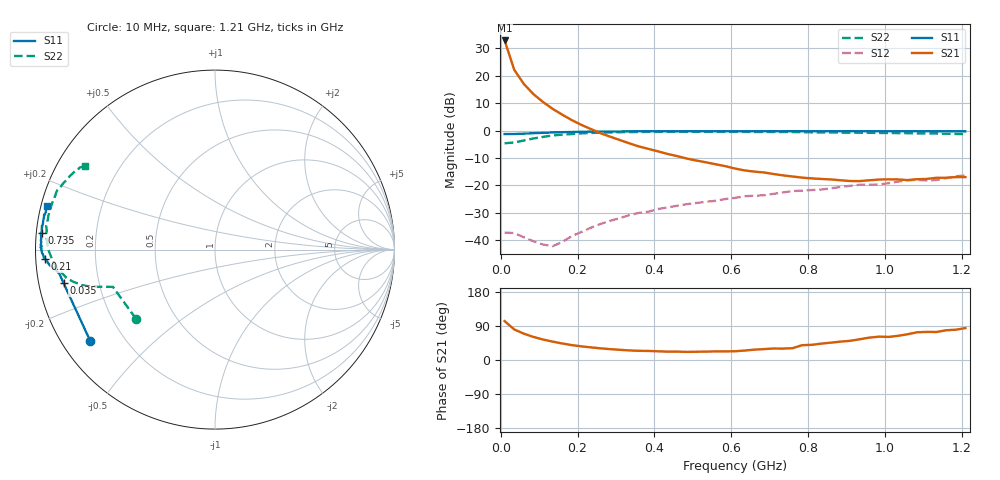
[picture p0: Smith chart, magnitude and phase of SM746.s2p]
!  POLYFET RF DEVICES
!  SM746
!  S PARAMETERS
!  VDS=50V, IDQ=600mA
# MHZ S MA R 50
! Freq=Mhz Mag[s11] Ang[s11] Mag[s21] Ang[s21] Mag[s12] Ang[s12] Mag[s22] Ang[s22]
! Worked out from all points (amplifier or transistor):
!   49 points, 10 MHz to 1.21 GHz, reference 50 ohm
!   highest |S21| = 32.8 dB at 10 MHz (marker M1)
!   |S21| within 3 dB of that: start of sweep to 17.04 MHz
!   unconditionally stable (mu >= 1): 121.7 MHz to 173.5 MHz; 679.3 MHz to end of sweep
!   at 210 MHz: K = 0.84, MSG = 19.5 dB, |S12| = -36.9 dB
!   at 610 MHz: K = 0.88, MSG = 5.3 dB, |S12| = -24.5 dB
!   at 1.21 GHz: K = 1.04, MAG = -1.6 dB, |S12| = -16.3 dB
!   S11 on the Smith chart (normalised r, x): 10 MHz: 0.08, -0.33; 35 MHz: 0.07, -0.11; 210 MHz: 0.03, -0.03; 735 MHz: 0.01, +0.05; 1.21 GHz: 0.02, +0.13
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10  0.862 -143.6  43.58 102.6  0.01389 14.4  0.585 -138.8
35  0.8641 -167.5  12.79 80.7  0.01359 2.3  0.6053 -159.9
60  0.8772 -171.1  7.042 69.4  0.01141 1.0  0.6581 -161.7
85  0.894 -172.7  4.602 60.9  0.00962 4.3  0.7161 -163.1
110  0.9078 -173.6  3.302 54.0  0.00841 22.7  0.7664 -165.0
135  0.9225 -174.4  2.483 48.5  0.00785 43.2  0.8116 -167.3
160  0.932 -175.3  1.946 43.6  0.00932 63.2  0.842 -169.2
185  0.9402 -176.2  1.546 39.3  0.01201 72.6  0.8631 -171.3
210  0.9472 -176.8  1.266 36.0  0.01423 79.7  0.8878 -173.4
260  0.9568 -178.0  0.8921 30.7  0.01993 87.4  0.9138 -177.4
285  0.9597 -178.5  0.7723 28.7  0.02276 88.1  0.9246 -179.3
335  0.9644 -179.1  0.5836 25.3  0.02883 90.0  0.935 177.6
410  0.9726 179.2  0.4167 23.0  0.03735 89.0  0.9438 173.4
485  0.9722 178.5  0.3082 21.4  0.04572 88.7  0.9461 169.8
610  0.9708 176.7  0.203 23.1  0.05935 90.1  0.9443 164.7
735  0.9705 174.6  0.1525 30.1  0.07458 90.9  0.9404 160.1
810  0.9687 174.5  0.1344 40.0  0.08249 89.1  0.9264 157.5
910  0.9739 172.3  0.1204 50.6  0.09835 90.0  0.913 154.7
1010  0.9705 170.6  0.1294 60.9  0.1098 91.2  0.9009 152.2
1060  0.9709 168.8  0.125 68.1  0.1242 88.6  0.894 150.7
1135  0.9682 168.2  0.138 73.9  0.1258 89.6  0.8807 148.7
1210  0.9665 165.3  0.1418 84.2  0.1527 87.8  0.8621 147.2
